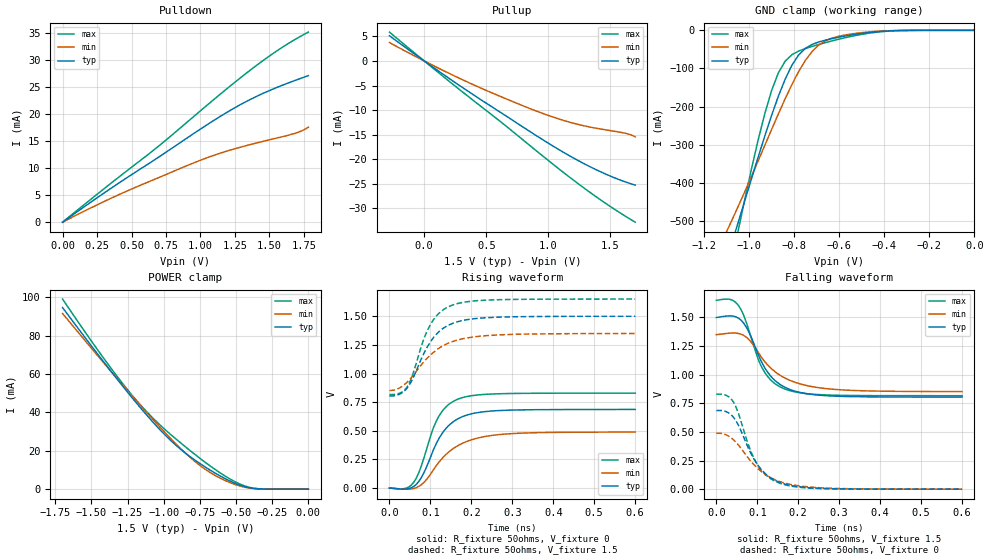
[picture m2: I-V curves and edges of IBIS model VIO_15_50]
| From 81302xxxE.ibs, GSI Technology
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[Model]   VIO_15_50
Model_type   I/O
Polarity   Non-Inverting
Vinl  =   0.5500V
Vinh  =   0.9500V
Vmeas =   0.75v
Rref  =   50
|  variable   typ   min   max
C_comp   3.0pF   2.5pF   3.5pF
[Receiver Thresholds]
Vth = 0.75V
Vth_min = 0.68V
Vth_max = 0.825V
Threshold_sensitivity = 1.0
Reference_supply Ext_ref
Vinh_ac = +200mv
Vinh_dc = +100mv
Vinl_ac = -200mv
Vinl_dc = -100mv
Tslew_ac = 550ps
|  variable   typ   min   max
[External Reference]   0.75   0.68   0.825
|  variable   typ   min   max
[Temperature Range]   50   100   0
|  variable   typ   min   max
[Voltage Range]   1.5   1.35   1.65
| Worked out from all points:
|   slope of the pulldown table from 0 to 0.225 V, typ, clamps not added: 55.3 ohm
|   slope of the pullup table from 0 to 0.225 V, typ, clamps not added: 56.6 ohm
|   GND clamp passes 1 mA (typ) near -0.36 V on its own axis
|   POWER clamp passes 1 mA (typ) near -0.42 V on its own axis
|   rising waveform, R_fixture 50ohms, V_fixture 0: 20-80 % time 61.2ps typ, 83ps min, 52.4ps max; typ from 0 V to 0.686 V
|   rising waveform, R_fixture 50ohms, V_fixture 1.5: 20-80 % time 64.2ps typ, 84.3ps min, 54.3ps max; typ from 0.805 V to 1.5 V
|   falling waveform, R_fixture 50ohms, V_fixture 1.5: 20-80 % time 64ps typ, 86.7ps min, 55.1ps max; typ from 1.5 V to 0.805 V
|   falling waveform, R_fixture 50ohms, V_fixture 0: 20-80 % time 63.8ps typ, 81.5ps min, 56ps max; typ from 0.686 V to 0 V
[Pullup]
| V(VDDQ-Vout)   typ   min   max
-280mV    5.117mA    3.738mA    5.862mA
40mV      -717.8uA   -514.8uA   -829.9uA
320mV     -5.603mA   -3.96mA    -6.529mA
560mV     -9.572mA   -6.647mA   -11.26mA
900mV     -15.14mA   -10.16mA   -18.2mA
1.12V     -18.55mA   -12.08mA   -22.63mA
1.32V     -21.31mA   -13.36mA   -26.44mA
1.48V     -23.2mA    -14.09mA   -29.27mA
1.62V     -24.59mA   -14.71mA   -31.56mA
1.7V      -25.26mA   -15.44mA   -32.79mA
[PullDown]
| voltage   typ   min   max
0V        -5.688nA   -12.79nA   -2.55nA
270mV     4.867mA    3.451mA    5.58mA
504mV     8.871mA    6.187mA    10.26mA
702mV     12.15mA    8.318mA    14.22mA
954mV     16.49mA    11.02mA    19.65mA
1.188V    20.3mA     13.15mA    24.67mA
1.35V     22.61mA    14.31mA    27.97mA
1.512V    24.53mA    15.34mA    31.02mA
1.692V    26.33mA    16.53mA    33.97mA
1.782V    27.17mA    17.6mA     35.24mA
[POWER Clamp]
|V(VDDQ-Vout)   typ   min   max
-1.7V     94.64mA    91.58mA    99.09mA
-1.428V   67.54mA    66.99mA    69.55mA
-1.224V   48.12mA    49.01mA    49.38mA
-1.122V   38.97mA    40.27mA    40.69mA
-986mV    27.88mA    29.06mA    30.72mA
-816mV    16.83mA    16.48mA    19.99mA
-714mV    11.58mA    10.4mA     14.03mA
-646mV    8.438mA    7.201mA    10.33mA
-544mV    4.31mA     3.482mA    5.399mA
-442mV    1.34mA     1.042mA    1.733mA
-340mV    155.8uA    132.4uA    187.3uA
0V        29.97nA    53.04nA    12.57nA
[GND Clamp]
|(Vout)   typ   min   max
-1.5V     -1.259A    -998.1mA   -1.702A
-1.11V    -621.1mA   -540.5mA   -701.3mA
-1.08V    -564.5mA   -502.7mA   -615.1mA
-1.05V    -506.9mA   -463.9mA   -529.8mA
-930mV    -276.8mA   -301.4mA   -218mA
-900mV    -223mA     -260.1mA   -157.9mA
-870mV    -172.8mA   -219.3mA   -111.5mA
-810mV    -91.52mA   -142.2mA   -63.98mA
-720mV    -36.91mA   -55.08mA   -42.14mA
-630mV    -21.51mA   -20.02mA   -27.42mA
-390mV    -1.861mA   -1.298mA   -2.48mA
0V        -7.463nA   -15.47nA   -3.343nA
[Ramp]
| voltage   typ   min   max
dV/dt_r   0.54/186p   0.48/213p   0.60/209p
dV/dt_f   0.86/129p   0.66/166p   1.07/101p
R_load  =   50ohms
[Rising Waveform]
R_fixture =   50ohms
V_fixture =   0
| Time   V(typ)   V(min)   V(max)
0s        148nV      384.4nV    62.25nV
36ps      -9.245mV   -9.202mV   -5.346mV
60ps      15.38mV    -3.41mV    53.82mV
84ps      133.1mV    49.26mV    261.4mV
108ps     339.4mV    162.8mV    532.2mV
120ps     427.8mV    222.2mV    622.9mV
144ps     543.5mV    312.6mV    728.5mV
168ps     606.2mV    372mV      777.3mV
288ps     679.4mV    472.6mV    824.8mV
600ps     686.3mV    488.6mV    828.8mV
[Rising Waveform]
R_fixture =   50ohms
V_fixture =   1.5
V_fixture_min =  1.35
V_fixture_max =  1.65
| Time   V(typ)   V(min)   V(max)
0s        804.6mV    852.4mV    816.7mV
24ps      817.8mV    872.6mV    827mV
42ps      867.5mV    920.1mV    876.3mV
54ps      933.8mV    966.1mV    961.9mV
84ps      1.175V     1.102V     1.302V
102ps     1.287V     1.167V     1.439V
120ps     1.363V     1.219V     1.523V
150ps     1.431V     1.274V     1.592V
264ps     1.492V     1.336V     1.644V
600ps     1.5V       1.349V     1.65V
[Falling Waveform]
R_fixture =   50ohms
V_fixture =   1.5
V_fixture_min = 1.35
V_fixture_max = 1.65
| Time   V(typ)   V(min)   V(max)
0s        1.5V       1.35V      1.65V
36ps      1.514V     1.364V     1.656V
54ps      1.494V     1.361V     1.605V
78ps      1.384V     1.313V     1.406V
102ps     1.179V     1.197V     1.138V
114ps     1.088V     1.134V     1.046V
138ps     967.6mV    1.042V     936.8mV
168ps     889.3mV    970.2mV    874.3mV
288ps     813.2mV    872mV      821mV
600ps     804.6mV    852.7mV    816.7mV
[Falling Waveform]
R_fixture =   50ohms
V_fixture =   0
| Time   V(typ)   V(min)   V(max)
0s        686.5mV    488.9mV    828.8mV
24ps      677.6mV    474.5mV    820.2mV
42ps      628mV      431.4mV    760.4mV
54ps      558.5mV    385.5mV    663.1mV
84ps      314.7mV    245.4mV    333.6mV
102ps     206.5mV    178.3mV    204.8mV
126ps     116.4mV    113.8mV    108.9mV
156ps     57.7mV     65.47mV    50.68mV
276ps     4.891mV    8.677mV    3.283mV
600ps     22.39uV    89.08uV    5.871uV
